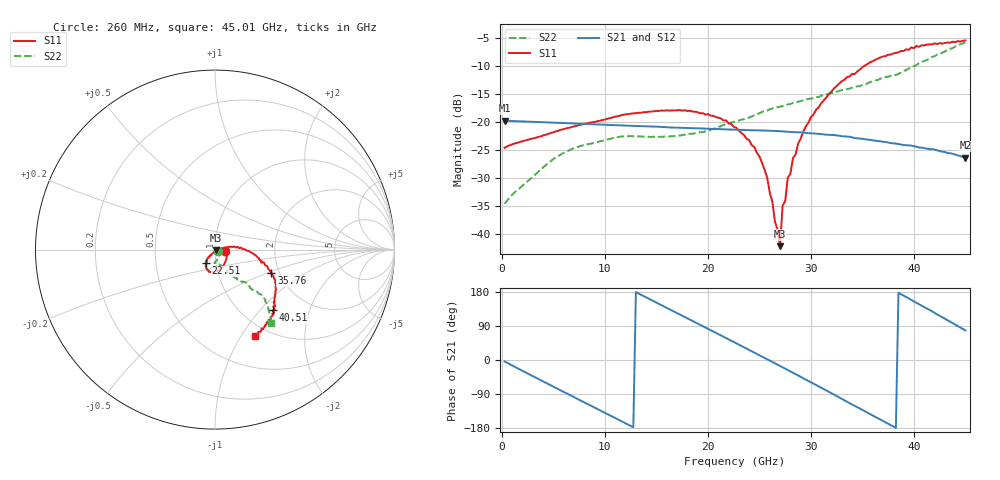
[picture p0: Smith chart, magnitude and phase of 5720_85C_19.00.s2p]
! Device:  ADRF5720
! Description: 0.5dB LSB GaAs MMIC 6-bit Digital Attenuator
! Frequency:  0.000009 -  40 GHz
! Ports:
!	RF1	= Port 1
!	RF2	= Port 2
! Vdd:  3.3 Volt
! Vss:  -3.3 Volt
! Control:  0/3.3 Volt
! State:  19.00 dB attenuation
! Data:  The device was measured using G-S-G Probes on a matrix board.
!  Data was collected using an calibrated 4 port network analyzer.
!  The reference plane for this measurement is at the launchers.
! Note:  Analog Devices supplies this data as a sample of measured data
!  for this product.  Your particular data for this product may vary.
!  Data was taken at 85 degrees C.
!  Analog Devices reserves the right to change this data at anytime.
# GHZ S DB R 45.0
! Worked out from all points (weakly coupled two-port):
!   180 points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, 260 MHz to 45.01 GHz, reference 45 ohm
!   highest |S21| = -19.78 dB at 260 MHz (marker M1); lowest = -26.4 dB at 45.01 GHz (marker M2)
!   lowest |S11| = -42.1 dB at 27.01 GHz (marker M3), VSWR 1.02, Z = 45.6 - j0.367 ohm
!   |S11| at or under -10 dB: start of sweep to 35.23 GHz
!   |S22| runs from -34.6 to -5.8 dB; largest |S21 - S12| = 0.00052
!   S11 on the Smith chart (normalised r, x): 260 MHz: 1.12, -0.02; 22.51 GHz: 0.90, -0.14; 35.76 GHz: 1.82, -0.53; 40.51 GHz: 1.36, -1.18; 45.01 GHz: 0.86, -1.16
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0.26  -24.60 -9.0  -19.78 -3.9  -19.77 -3.9  -34.56 -25.7
4.76  -21.98 -37.2  -20.11 -67.1  -20.09 -67.0  -26.94 -65.2
7.76  -20.47 -56.8  -20.33 -108.5  -20.32 -108.5  -24.22 -81.3
15.26  -18.04 -94.4  -20.87 147.9  -20.85 148.0  -22.63 -91.2
20.01  -18.61 -113.2  -21.20 82.3  -21.19 82.4  -21.55 -74.9
22.51  -20.89 -123.3  -21.37 47.6  -21.36 47.8  -19.98 -66.9
22.76  -21.03 -123.0  -21.39 44.1  -21.37 44.3  -19.88 -67.1
24.51  -24.46 -128.6  -21.49 19.8  -21.48 20.1  -18.83 -64.6
25.51  -28.50 -124.1  -21.53 5.7  -21.52 5.9  -18.04 -63.5
26.26  -34.16 -116.4  -21.60 -5.1  -21.58 -4.8  -17.63 -61.6
26.51  -37.68 -104.5  -21.62 -8.6  -21.60 -8.3  -17.44 -61.0
27.01  -42.10 -30.8  -21.65 -15.8  -21.63 -15.5  -17.28 -60.0
27.26  -34.87 -9.2  -21.69 -19.4  -21.68 -19.2  -17.16 -60.4
27.51  -34.10 6.9  -21.72 -22.9  -21.71 -22.7  -17.09 -59.5
27.76  -29.91 6.0  -21.75 -26.5  -21.73 -26.2  -16.88 -60.2
28.76  -23.91 11.5  -21.85 -40.6  -21.84 -40.3  -16.41 -59.6
30.26  -18.68 5.8  -22.04 -62.4  -22.03 -62.1  -15.81 -58.3
33.01  -12.75 -8.2  -22.55 -102.6  -22.53 -102.4  -14.34 -54.6
35.76  -9.38 -22.4  -23.20 -142.8  -23.18 -142.5  -12.91 -51.2
37.76  -8.03 -31.8  -23.77 -171.9  -23.75 -171.6  -11.79 -46.9
40.51  -6.63 -46.5  -24.55 147.1  -24.53 147.5  -9.52 -45.0
45.01  -5.51 -64.9  -26.35 78.0  -26.32 78.4  -5.82 -52.8
